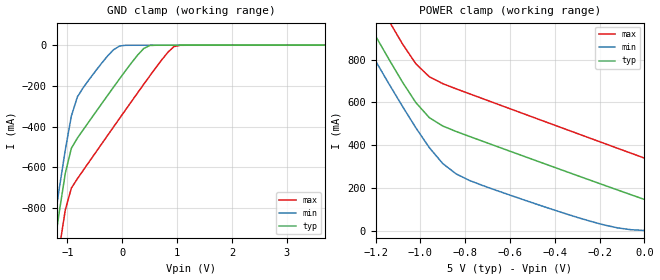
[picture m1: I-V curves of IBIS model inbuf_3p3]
| IBIS file logicTx.ibs created by s2ibis3 verion 1.1
| North Carolina State University, ERL, 2006
[IBIS ver] 4.0
[File name] f0480-inbuf3p3.ibs
[File Rev] 0.1
[Date]  April 14, 2016
[Source] Integrated Device Technology, Inc.
|   Component dummycomp
[Component] F0480
[Manufacturer] Integrated Device Technology, Inc.
[Package]
| variable   typ   min   max
R_pkg   2.0000m   1.0000m   4.0000m
L_pkg   0.2000nH   0.1000nH   0.4000nH
C_pkg   2.0000pF   1.0000pF   4.0000pF
[Pin]  signal_name   model_name   R_pin   L_pin   C_pin
5   VDD   POWER
4   CLMP_VDD   POWER
3   CLMP_GND   GND
2   net1   inbuf_3p3
1   gnd   GND
[Pin Mapping]  pulldown_ref   pullup_ref   gnd_clamp_ref   power_clamp_ref
5   NC   DRV_VDD   NC   NC
4   NC   CLMP_VDD   NC   NC
3   CLMP_GND   NC   NC   NC
2   NC   NC   CLMP_GND   CLMP_VDD
1   DRV_GND   NC   NC   NC
| Models and submodels in the file (1): inbuf_3p3 (Input)
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|   Model inbuf_3p3
[Model]  inbuf_3p3
Model_type Input
Polarity   Non-Inverting
Vinl =   1.1550V
Vinh =   2.1450V
C_comp   4.2734pF   4.1666pF   4.3090pF
[Temperature Range]   25.0000   0.1250k   0.0
[Pullup Reference]   2.5000V   2.2500V   2.7500V
[Pulldown Reference]   0.0V   0.0V   0.0V
[POWER Clamp Reference]   5.0000V   4.5000V   5.5000V
[GND Clamp Reference]   0.0V   0.0V   0.0V
[GND_clamp]
|Voltage   I(typ)   I(min)   I(max)
|  0.0000   -0.1463A   -1.1906mA   -0.3396A
-5V       -8.599A    -8.352A    -8.888A
-1.26V    -1.022A    -904.1mA   -1.206A
-1.15V    -818.7mA   -703.6mA   -998.8mA
-1.04V    -628.6mA   -513.8mA   -808.3mA
-930mV    -506.1mA   -348mA     -701.6mA
-820mV    -455.9mA   -253.8mA   -655.4mA
-270mV    -246.7mA   -53.09mA   -443.1mA
-50mV     -164.7mA   -3.86mA    -358.7mA
390mV     -15.99mA   -27.45nA   -191.7mA
940mV     -509.1pA   -1.587nA   -6.909mA
4.46V     305.4uA    443.5uA    266.7uA
4.79V     71.33mA    59.38mA    74.71mA
[POWER_clamp]
|Voltage   I(typ)   I(min)   I(max)
-4.92V    8.435A     8.19A      8.722A
-1.32V    1.137A     1.016A     1.322A
-1.26V    1.022A     904.1mA    1.206A
-1.2V     910.1mA    793.8mA    1.092A
-1.14V    800.7mA    685.9mA    980.5mA
-1.08V    694.8mA    581.3mA    873.3mA
-1.02V    598.5mA    480.8mA    780.1mA
-960mV    528.5mA    388.2mA    719.7mA
-900mV    489.5mA    313.9mA    687.5mA
-840mV    463.8mA    265.3mA    663.2mA
-300mV    258mA      62.57mA    454.7mA
0V        146.3mA    1.191mA    339.6mA
